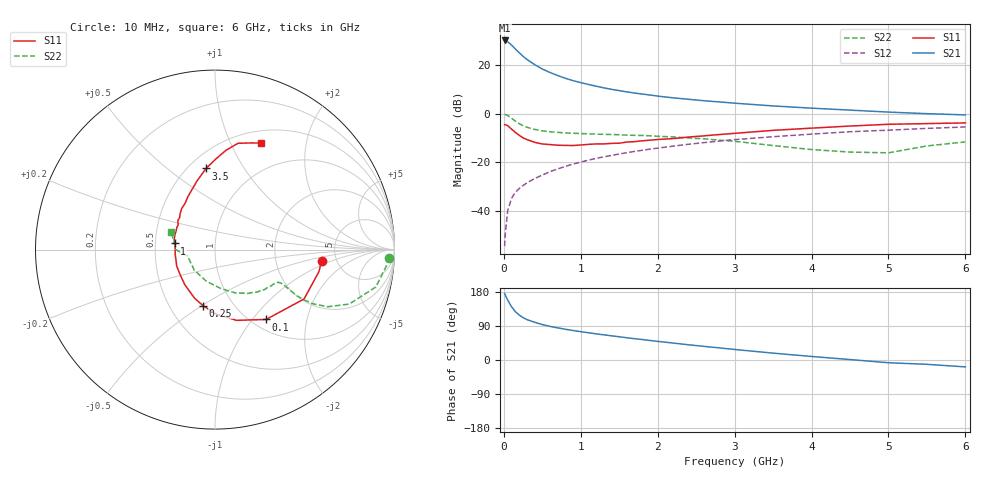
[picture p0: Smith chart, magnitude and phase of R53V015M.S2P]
! SIEMENS Small Signal Semiconductors
! BFR183
! Si NPN RF Bipolar Junction Transistor in SOT23
! VCE = 3 V  IC = 15 mA
! Common Emitter S-Parameters:  May  1996
# GHz  S  MA  R  50
!  f  S11  S21  S12  S22
! GHz  MAG  ANG  MAG  ANG  MAG  ANG  MAG  ANG
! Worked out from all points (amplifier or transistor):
!   36 points, 10 MHz to 6 GHz, reference 50 ohm
!   highest |S21| = 30.1 dB at 10 MHz (marker M1)
!   |S21| within 3 dB of that: start of sweep to 134.2 MHz
!   unconditionally stable (mu >= 1): 640.7 MHz to 2.406 GHz
!   at 250 MHz: K = 0.74, MSG = 26.6 dB, |S12| = -29.5 dB
!   at 1.4 GHz: K = 1.05, MAG = 12.2 dB, |S12| = -17.1 dB
!   at 6 GHz: K = 0.89, MSG = 2.5 dB, |S12| = -5.5 dB
!   S11 on the Smith chart (normalised r, x): 10 MHz: 3.80, -0.76; 100 MHz: 1.16, -1.17; 250 MHz: 0.73, -0.51; 1 GHz: 0.63, +0.05; 3.5 GHz: 0.61, +0.69; 6 GHz: 0.64, +1.31
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0.01  0.597 -6.2  31.93 175.3  0.0019 86.4  0.9709 -2.6
0.02  0.592 -12.0  31.49 170.6  0.0036 85.1  0.959 -5.5
0.05  0.5673 -29.0  30.01 158.1  0.0102 79.1  0.9198 -13.1
0.1  0.4822 -53.8  25.77 140.6  0.0182 71.4  0.807 -22.1
0.15  0.4123 -73.0  21.27 127.5  0.0244 67.1  0.7037 -26.9
0.2  0.3601 -88.9  17.85 118.6  0.029 66.1  0.6252 -28.9
0.25  0.3193 -102.0  15.09 111.8  0.0334 65.9  0.5653 -29.5
0.3  0.2938 -112.8  13.02 106.7  0.0379 66.5  0.5266 -29.4
0.4  0.258 -130.7  10.2 99.6  0.0465 67.1  0.4756 -28.5
0.5  0.2386 -145.0  8.278 93.5  0.0549 68.6  0.4429 -27.5
0.6  0.2322 -156.8  7.011 88.8  0.0643 69.0  0.4257 -27.0
0.7  0.2248 -165.5  6.077 84.8  0.0736 69.5  0.4134 -26.9
0.8  0.2232 -173.7  5.336 81.1  0.0827 69.0  0.4038 -27.1
1  0.2274 171.3  4.342 74.7  0.1014 68.5  0.3912 -28.0
1.1  0.2345 165.6  3.982 71.9  0.1111 68.2  0.3858 -29.2
1.3  0.2394 155.1  3.392 66.4  0.13 66.8  0.3763 -31.0
1.6  0.262 142.3  2.802 58.6  0.1582 64.2  0.3629 -35.1
2.2  0.3077 122.7  2.117 44.7  0.2155 58.4  0.3337 -45.1
3.5  0.4547 96.3  1.443 18.1  0.3367 42.6  0.2214 -80.5
4.5  0.5573 83.6  1.184 1.2  0.4258 30.1  0.1627 -135.2
5.5  0.6258 71.7  1.001 -11.4  0.499 18.2  0.2176 -179.9
6  0.6468 66.7  0.944 -18.2  0.5336 10.6  0.2634 157.6
